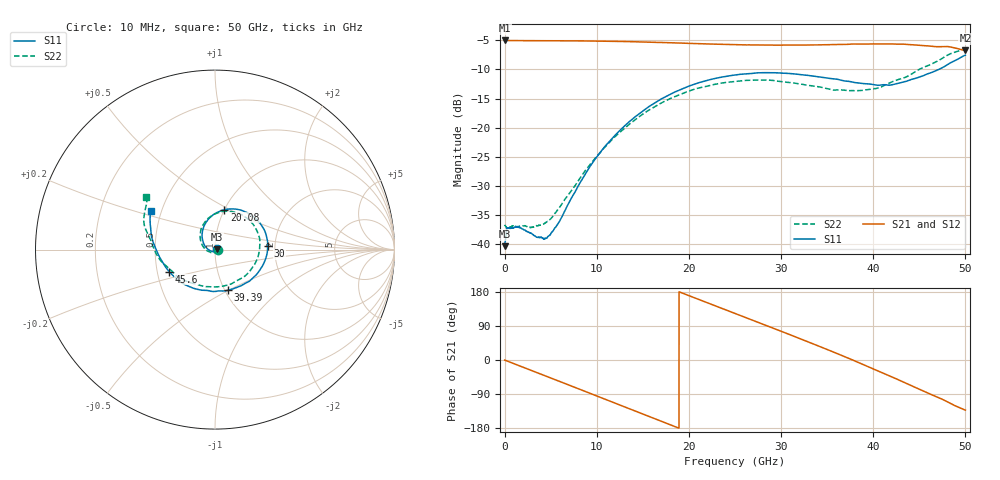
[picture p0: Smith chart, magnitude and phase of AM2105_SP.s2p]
!Keysight Technologies,N5245B,MY58422270,A.16.20.02
!Date: Wednesday, March 11, 2026 23:37:45
!Correction: S11(C  2-Port  )
!S21(C  2-Port  )
!S12(C  2-Port  )
!S22(C  2-Port  )
!S2P File: Measurements: S11, S21, S12, S22:
# Hz S  dB  R 50
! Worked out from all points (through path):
!   6401 points, 10 MHz to 50 GHz, reference 50 ohm
!   highest |S21| = -5.03 dB at 10 MHz (marker M1); lowest = -6.7 dB at 50 GHz (marker M2)
!   group delay of S21, straight-line fit = 27 ps
!   lowest |S11| = -40.3 dB at 10 MHz (marker M3), VSWR 1.02, Z = 51 + j0.19 ohm
!   |S11| at or under -10 dB: start of sweep to 47.1 GHz
!   |S22| runs from -37.3 to -6.4 dB; largest |S21 - S12| = 0.0072
!   S11 on the Smith chart (normalised r, x): 10 MHz: 1.02, +0.00; 20.08 GHz: 1.00, +0.47; 30 GHz: 1.83, +0.07; 39.39 GHz: 1.03, -0.50; 45.6 GHz: 0.58, -0.15; 50 GHz: 0.44, +0.23
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1e7  -40.34 11.2  -5.03 -0.3  -5.09 -0.9  -36.69 -17.2
4.317906e8  -37.19 -2.2  -5.04 -4.1  -5.05 -4.1  -37.20 -5.4
1.212884e9  -37.07 -12.3  -5.05 -11.5  -5.05 -11.5  -36.97 -15.2
4.704373e9  -38.67 -92.4  -5.07 -44.5  -5.07 -44.5  -36.06 -92.0
5.92288e9  -36.19 -131.6  -5.08 -56.0  -5.09 -56.0  -33.80 -122.4
8.34427e9  -29.07 -178.2  -5.11 -79.0  -5.11 -79.0  -28.31 -164.0
1.221068e10  -20.94 141.2  -5.19 -115.9  -5.19 -115.9  -21.23 152.9
1.455397e10  -17.68 121.1  -5.26 -138.3  -5.27 -138.3  -18.18 131.7
1.667854e10  -15.38 103.7  -5.37 -158.5  -5.37 -158.5  -16.05 113.2
2.00763e10  -12.82 76.8  -5.53 169.2  -5.53 169.2  -13.67 84.9
2.234147e10  -11.74 59.4  -5.64 147.8  -5.65 147.9  -12.73 66.5
2.5005e10  -10.96 39.8  -5.75 123.0  -5.75 123.0  -12.06 45.0
2.748107e10  -10.59 21.9  -5.81 99.7  -5.81 99.7  -11.82 24.3
3.0004e10  -10.62 3.6  -5.82 76.0  -5.83 75.9  -12.08 1.7
3.333927e10  -11.12 -20.4  -5.80 43.9  -5.80 43.9  -12.82 -30.6
3.651051e10  -11.84 -45.5  -5.70 12.8  -5.70 12.8  -13.52 -66.4
3.939275e10  -12.48 -72.6  -5.65 -16.7  -5.64 -16.7  -13.45 -103.8
4.167354e10  -12.71 -98.8  -5.63 -40.8  -5.62 -40.7  -12.38 -133.8
4.356379e10  -12.05 -123.6  -5.69 -61.5  -5.70 -61.5  -11.30 -155.7
4.560244e10  -10.95 -154.3  -5.93 -83.5  -5.93 -83.5  -9.55 -177.7
4.791448e10  -9.32 174.9  -6.06 -108.7  -6.07 -108.7  -7.66 161.7
5e10  -7.57 149.2  -6.73 -132.3  -6.81 -131.7  -6.35 142.5
